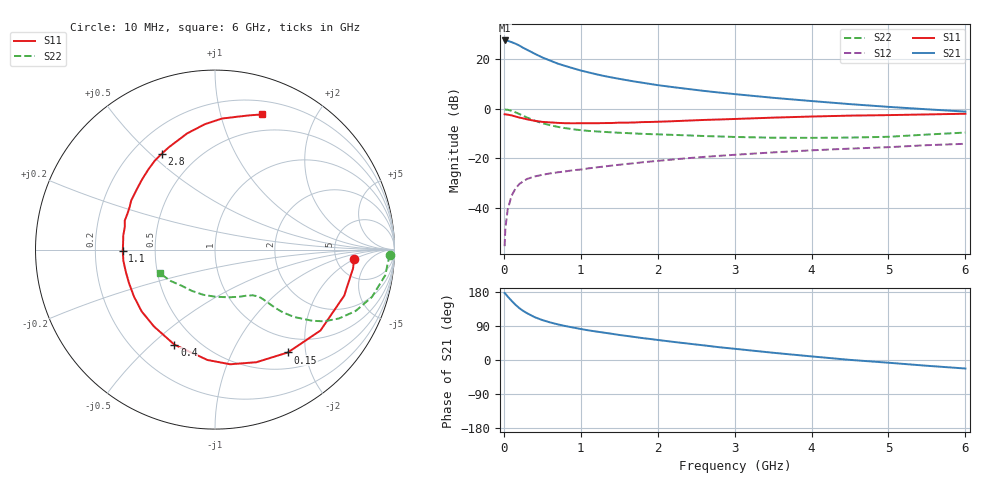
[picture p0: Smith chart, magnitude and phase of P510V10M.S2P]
! SIEMENS Small Signal Semiconductors
! BFP183
! Si NPN RF Bipolar Junction Transistor in SOT143
! VCE = 10 V  IC = 10 mA
! Common Emitter S-Parameters:  March  1996
# GHz  S  MA  R  50
!  f  S11  S21  S12  S22
! GHz  MAG  ANG  MAG  ANG  MAG  ANG  MAG  ANG
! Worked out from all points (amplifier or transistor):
!   36 points, 10 MHz to 6 GHz, reference 50 ohm
!   highest |S21| = 27.6 dB at 10 MHz (marker M1)
!   |S21| within 3 dB of that: start of sweep to 253.7 MHz
!   unconditionally stable (mu >= 1): 1.295 GHz to 5.734 GHz
!   at 250 MHz: K = 0.30, MSG = 27.0 dB, |S12| = -29.3 dB
!   at 1.4 GHz: K = 1.03, MAG = 16.8 dB, |S12| = -22.9 dB
!   at 6 GHz: K = 0.96, MSG = 6.5 dB, |S12| = -14.1 dB
!   S11 on the Smith chart (normalised r, x): 10 MHz: 7.46, -1.94; 150 MHz: 0.74, -1.68; 400 MHz: 0.37, -0.59; 1.1 GHz: 0.32, -0.01; 2.8 GHz: 0.32, +0.54; 6 GHz: 0.33, +1.36
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0.01  0.7771 -3.8  24.01 177.0  0.0017 75.7  0.9768 -1.7
0.02  0.7762 -7.8  23.95 175.1  0.0039 78.6  0.9686 -3.4
0.05  0.7643 -19.6  23.67 167.5  0.0093 79.4  0.9591 -8.6
0.1  0.7406 -37.5  22.21 156.4  0.0176 70.3  0.9134 -16.8
0.15  0.7022 -54.7  20.73 146.0  0.0245 63.8  0.8548 -23.6
0.2  0.6686 -69.8  19.02 137.1  0.0304 58.3  0.7895 -29.1
0.25  0.6444 -82.5  17.11 129.8  0.0344 53.3  0.7279 -33.3
0.3  0.6164 -93.9  15.61 123.7  0.0385 49.9  0.6713 -36.2
0.4  0.5759 -113.1  13 113.1  0.0433 45.9  0.5796 -40.4
0.5  0.5469 -128.4  10.9 105.4  0.0468 42.4  0.5139 -42.8
0.6  0.5344 -139.9  9.449 99.3  0.0499 41.5  0.469 -44.0
0.7  0.5217 -150.0  8.193 94.1  0.0525 40.9  0.4339 -44.7
0.9  0.5121 -165.9  6.597 85.7  0.0579 40.9  0.3878 -45.8
1.1  0.5141 -178.9  5.451 78.2  0.0631 41.2  0.3596 -47.0
1.5  0.5282 162.1  4.037 66.1  0.0746 41.2  0.3299 -50.5
1.8  0.5412 149.6  3.371 57.9  0.0836 41.6  0.3136 -54.5
2.2  0.5641 136.0  2.746 47.9  0.0953 40.3  0.2987 -61.0
2.8  0.6109 119.2  2.134 33.7  0.1129 37.1  0.2778 -73.0
3.5  0.6657 103.5  1.673 19.1  0.1325 32.9  0.2623 -90.1
4.5  0.731 87.0  1.247 0.3  0.1579 25.8  0.2638 -119.5
5.5  0.7726 75.5  0.981 -15.2  0.1852 19.5  0.3035 -145.0
6  0.798 70.7  0.881 -22.5  0.1976 15.5  0.333 -156.5
